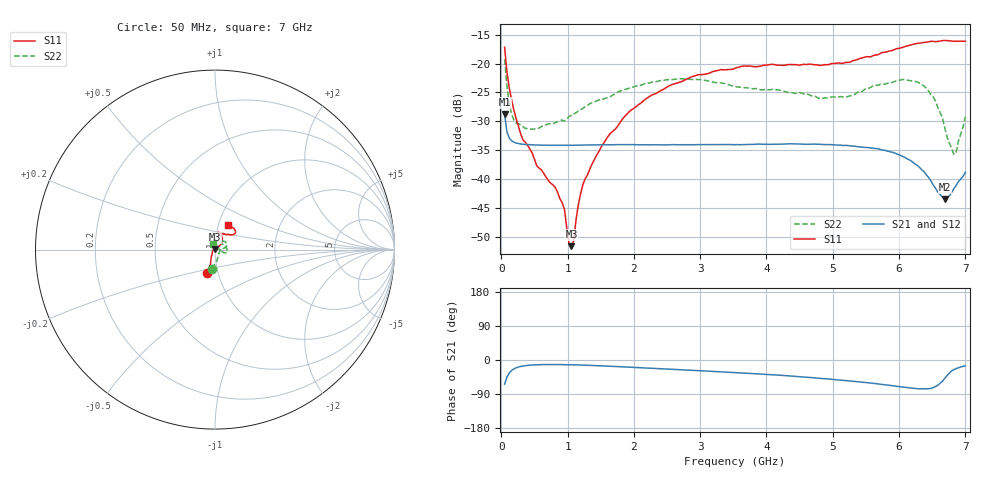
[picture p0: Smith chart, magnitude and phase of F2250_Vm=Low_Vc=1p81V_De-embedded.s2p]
! Integrated Device Technology
! Corporate Headquarters
! 6024 Silver Creek Valley Road
! San Jose, CA 95138  USA
! Phone:  1-408-284-8200
! Toll Free:  1-800-223-1366
! Webpage:  http://www.idt.com/
! Timing and RF Division
! 515 Groton Road, Suite 102
! Westford, MA 01886-6024
! Device:  F2250
! Description: Voltage Variable RF Attenuator
! Frequency:  50.0 -  6000.00 MHz
! Package:  3x3 mm Thin QFN Plastic Package: 16 pin
! Ports:  2 RF, 3 DC
!  Pin  1  = GND
!  Pin  2  = NC
!  Pin  3  = RF1  = Port 1
!  Pin  4  = NC
!  Pin  5  = GND
!  Pin  6  = GND
!  Pin  7  = GND
!  Pin  8  = GND
!  Pin  9  = NC
!  Pin 10  = RF2  = Port 2
!  Pin 11  = NC
!  Pin 12  = GND
!  Pin 13  = GND
!  Pin 14  = VCNTRL
!  Pin 15  = VDD
!  Pin 16  = VMODE
! Vcntrl:  1.810 Volts
! Vmode:  +0.000 Volts
! Vdd:  +3.30  Volts
! Current:  1.185 mA
! Data:  The device was measured on a the F2250 evaluation board which has
!  individual transmission lines to the RF pins.  Data was collected
!  using a calibrated network analyzer.  The evaluation board was
!  de-embedded using a TRL calibration technique.
!  The reference plane is the edge of the package pin.
! Misc:  SN 10
!  Action Tracker AT0258
! Date Measured:  2014-11-26
! Date:  2015-10-15  MJV
! Note:
!  Integrated Device Technology supplies this data as a sample of measured
!  data at the package pin for this product.  Your particular data for this
!  product may vary.
!  Data was taken at 25 degrees C.
!  Integrated Device Technology reserves the right to change this data at anytime.
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# GHz S dB R 50
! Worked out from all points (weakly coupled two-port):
!   201 points, 50 MHz to 7 GHz, reference 50 ohm
!   highest |S21| = -28.79 dB at 50 MHz (marker M1); lowest = -43.5 dB at 6.687 GHz (marker M2)
!   lowest |S11| = -51.7 dB at 1.058 GHz (marker M3), VSWR 1.01, Z = 49.9 + j0.233 ohm
!   |S11| at or under -10 dB: start of sweep to end of sweep
!   |S22| runs from -35.8 to -19.2 dB; largest |S21 - S12| = 6e-05
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0.05  -17.17 -108.4  -28.79 -63.8  -28.79 -63.8  -19.25 -98.9
0.1195  -24.20 -111.4  -32.90 -34.5  -32.90 -34.5  -26.87 -69.7
0.22375  -29.54 -121.5  -33.79 -20.7  -33.79 -20.7  -30.32 -45.6
0.5365  -37.75 -154.3  -34.13 -12.5  -34.13 -12.5  -31.34 -8.9
0.91875  -44.14 157.8  -34.18 -12.2  -34.18 -12.2  -29.79 -1.9
0.9535  -45.31 169.9  -34.18 -12.3  -34.18 -12.3  -30.01 0.1
1.023  -51.19 142.4  -34.18 -12.5  -34.17 -12.5  -29.17 2.0
1.05775  -51.66 116.6  -34.17 -12.6  -34.16 -12.6  -28.97 3.0
1.0925  -50.73 83.3  -34.16 -12.8  -34.16 -12.8  -28.79 2.8
1.162  -44.47 53.0  -34.16 -13.1  -34.15 -13.1  -28.24 2.4
1.2315  -40.95 41.6  -34.13 -13.4  -34.14 -13.4  -27.76 2.1
1.6485  -32.07 41.1  -34.09 -16.5  -34.09 -16.5  -25.71 10.3
2.37825  -24.87 47.0  -34.09 -22.8  -34.09 -22.9  -23.03 20.9
3.525  -20.83 72.3  -34.07 -33.2  -34.07 -33.2  -24.01 48.3
4.7065  -20.20 72.3  -33.97 -46.8  -33.96 -46.9  -25.66 54.5
5.22775  -19.81 56.2  -34.22 -54.9  -34.21 -54.9  -25.72 29.4
5.85325  -17.84 40.3  -35.27 -66.8  -35.26 -67.0  -23.32 -2.3
6.3745  -16.35 41.3  -38.74 -76.3  -38.76 -76.3  -23.87 -16.7
6.54825  -16.21 45.1  -41.60 -70.1  -41.61 -70.0  -26.50 -18.0
6.68725  -16.00 48.7  -43.53 -48.7  -43.52 -48.4  -31.09 -2.1
6.82625  -16.15 53.5  -41.70 -25.5  -41.68 -25.5  -35.77 48.5
7  -16.14 63.2  -38.85 -15.6  -38.81 -15.7  -29.19 106.7
